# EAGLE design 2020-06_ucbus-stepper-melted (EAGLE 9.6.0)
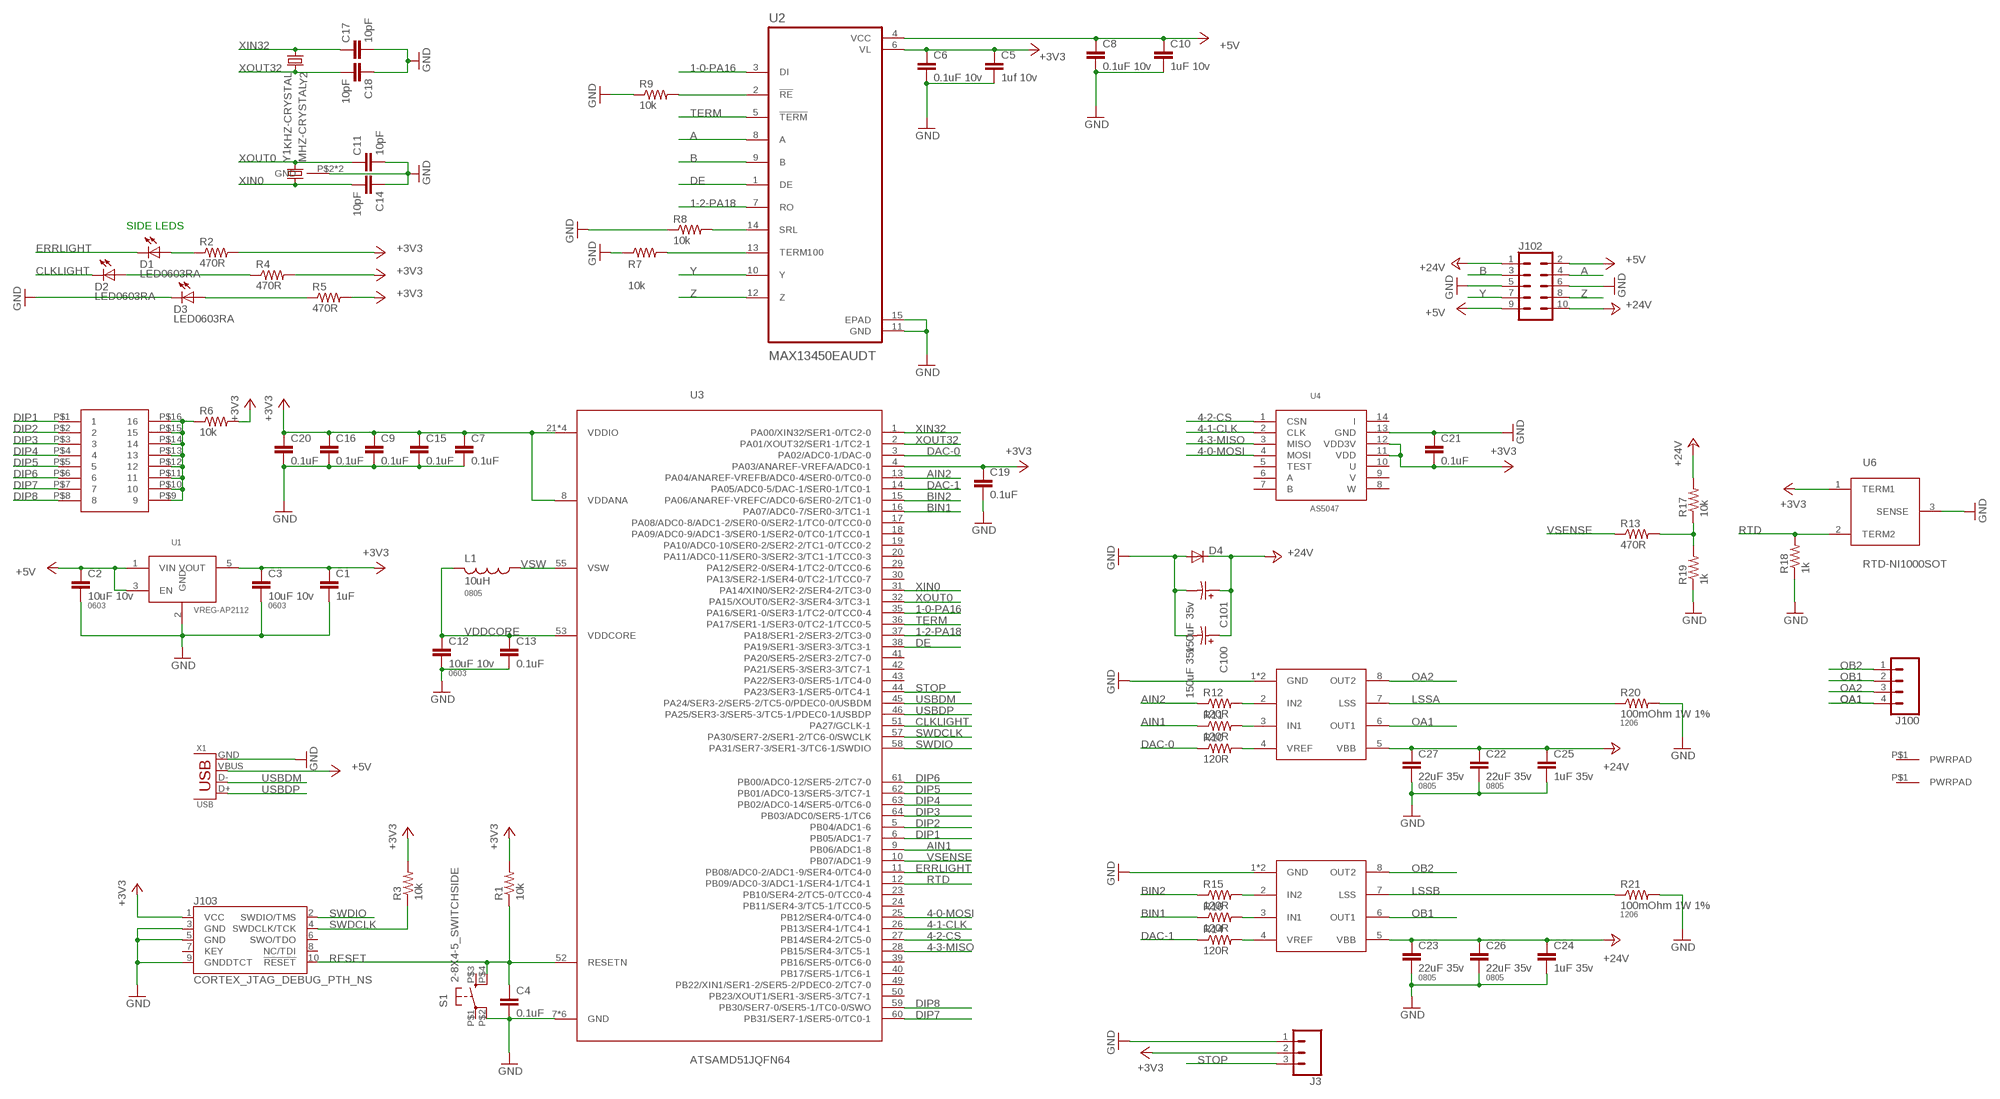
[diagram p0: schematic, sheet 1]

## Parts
C1  1uF  CAP0402  [0402]
C2  10uF 10v  CAP0603-CAP  [0603-CAP]
C3  10uF 10v  CAP0603-CAP  [0603-CAP]
C4  0.1uF  CAP0402  [0402]
C5  1uf 10v  CAP0402  [0402]
C6  0.1uF 10v  CAP0402  [0402]
C7  0.1uF  CAP0402  [0402]
C8  0.1uF 10v  CAP0402  [0402]
C9  0.1uF  CAP0402  [0402]
C10  1uF 10v  CAP0402  [0402]
C11  10pF  CAP0402  [0402]
C12  10uF 10v  CAP0603-CAP  [0603-CAP]
C13  0.1uF  CAP0402  [0402]
C14  10pF  CAP0402  [0402]
C15  0.1uF  CAP0402  [0402]
C16  0.1uF  CAP0402  [0402]
C17  10pF  CAP0402  [0402]
C18  10pF  CAP0402  [0402]
C19  0.1uF  CAP0402  [0402]
C20  0.1uF  CAP0402  [0402]
C21  0.1uF  CAP0402  [0402]
C22  22uF 35v  CAP0805  [0805]
C23  22uF 35v  CAP0805  [0805]
C24  1uF 35v  CAP0402  [0402]
C25  1uF 35v  CAP0402  [0402]
C26  22uF 35v  CAP0805  [0805]
C27  22uF 35v  CAP0805  [0805]
C100  150uF 35v  CAP-POLCAP_POL_SMD6.6X6.6  [SMD-ELEC-CAP]
C101  150uF 35v  CAP-POLCAP_POL_SMD6.6X6.6  [SMD-ELEC-CAP]
D1  LED0603RA  [LED0603-RIGHTANGLE]
D2  LED0603RA  [LED0603-RIGHTANGLE]
D3  LED0603RA  [LED0603-RIGHTANGLE]
D4  DIODESMA403D  [SMA-403D]
J1  PWRPADM3-SKINNY  [PWRPAD_3-25MM-SKINNY]
J2  PWRPADM3-SKINNY  [PWRPAD_3-25MM-SKINNY]
J3  CONN_03SMD_RA_MALE  [1X03_SMD_RA_MALE]
J100  CONN_04SCREW_LOCK  [SCREWTERMINAL-3.5MM-4_LOCK]
J101  DIPSWITCH-80100  [DIPSWITCH-8-0100]
J102  CONN_05X2SHD_LOCK_LATCH  [2X5-SHROUDED_LOCK_LATCH]
J103  CORTEX_JTAG_DEBUG_PTH_NS  [2X5-PTH-1.27MM-NO_SILK]
L1  10uH  INDUCTOR-0805  [0805]
R1  10k  RESISTOR0402  [0402]
R2  470R  RESISTOR0402  [0402]
R3  10k  RESISTOR0402  [0402]
R4  470R  RESISTOR0402  [0402]
R5  470R  RESISTOR0402  [0402]
R6  10k  RESISTOR0402  [0402]
R7  10k  RESISTOR0402  [0402]
R8  10k  RESISTOR0402  [0402]
R9  10k  RESISTOR0402  [0402]
R10  120R  RESISTOR0402  [0402]
R11  120R  RESISTOR0402  [0402]
R12  120R  RESISTOR0402  [0402]
R13  470R  RESISTOR0402  [0402]
R14  120R  RESISTOR0402  [0402]
R15  120R  RESISTOR0402  [0402]
R16  120R  RESISTOR0402  [0402]
R17  10k  RESISTOR0402  [0402]
R18  1k  RESISTOR0402  [0402]
R19  1k  RESISTOR0402  [0402]
R20  100mOhm 1W 1%  RESISTOR1206  [1206]
R21  100mOhm 1W 1%  RESISTOR1206  [1206]
S1  2-8X4-5_SWITCHSIDE  [TACT-SWITCH-SIDE]
U1  VREG-AP2112  [SOT23-5]
U2  MAX13450EAUDT  [SOP65P637X110-14N]
U3  ATSAMD51JQFN64  [QFN-64-9X9MM-SMALLPAD]
U4  AS5047  [TSSOP14]
U5  A4950  [SOIC8_PAD]
U6  RTD-NI1000SOT  [SOT23]
U7  A4950  [SOIC8_PAD]
X1  USB  [USB_MICRO_609-4613-1-ND]
Y1  MHZ-CRYSTAL  [4-SMD-3.2X2.5]
Y2  KHZ-CRYSTAL  [2-SMD-3.2X1.5MM]

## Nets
1-0-PA16: U2.3(DI) U3.35(PA16/SER1-0/SER3-1/TC2-0/TCC0-4)
1-2-PA18: U2.7(RO) U3.37(PA18/SER1-2/SER3-2/TC3-0)
4-0-MOSI: U3.25(PB12/SER4-0/TC4-0) U4.4(MOSI)
4-1-CLK: U3.26(PB13/SER4-1/TC4-1) U4.2(CLK)
4-2-CS: U3.27(PB14/SER4-2/TC5-0) U4.1(CSN)
4-3-MISO: U3.28(PB15/SER4-3/TC5-1) U4.3(MISO)
+3V3: C1.1 C3.1 C5.1 C6.1 C7.1 C9.1 C15.1 C16.1 C19.1 C20.1 C21.2 J3.2 J103.1(VCC) R1.2 R2.2 R3.2 R4.2 R5.2 R6.2 U1.5(VOUT) U2.6(VL) U3.4(PA03/ANAREF-VREFA/ADC0-1) U3.8(VDDANA) U3.21(VDDIO) U3.34(VDDIO) U3.48(VDDIO) U3.56(VDDIO) U4.11(VDD) U4.12(VDD3V) U6.1(TERM1)
+5V: C2.1 C8.1 C10.1 J102.2 J102.9 U1.1(VIN) U1.3(EN) U2.4(VCC) X1.VBUS
+24V: C22.1 C23.1 C24.1 C25.1 C26.1 C27.1 C100.A C101.A D4.P$1(C) J102.1 J102.10 R17.2 U5.5(VBB) U7.5(VBB)
A: J102.4 U2.8(A)
AIN1: R11.1 U3.9(PB06/ADC1-8)
AIN2: R12.1 U3.13(PA04/ANAREF-VREFB/ADC0-4/SER0-0/TC0-0)
B: J102.3 U2.9(B)
BIN1: R16.1 U3.16(PA07/ADC0-7/SER0-3/TC1-1)
BIN2: R15.1 U3.15(PA06/ANAREF-VREFC/ADC0-6/SER0-2/TC1-0)
CLKLIGHT: D2.2(C) U3.51(PA27/GCLK-1)
DAC-0: R10.1 U3.3(PA02/ADC0-1/DAC-0)
DAC-1: R14.1 U3.14(PA05/ADC0-5/DAC-1/SER0-1/TC0-1)
DE: U2.1(DE) U3.38(PA19/SER1-3/SER3-3/TC3-1)
DIP1: J101.P$1 U3.6(PB05/ADC1-7)
DIP2: J101.P$2 U3.5(PB04/ADC1-6)
DIP3: J101.P$3 U3.64(PB03/ADC0/SER5-1/TC6)
DIP4: J101.P$4 U3.63(PB02/ADC0-14/SER5-0/TC6-0)
DIP5: J101.P$5 U3.62(PB01/ADC0-13/SER5-3/TC7-1)
DIP6: J101.P$6 U3.61(PB00/ADC0-12/SER5-2/TC7-0)
DIP7: J101.P$7 U3.60(PB31/SER7-1/SER5-0/TC0-1)
DIP8: J101.P$8 U3.59(PB30/SER7-0/SER5-1/TC0-0/SWO)
ERRLIGHT: D1.2(C) U3.11(PB08/ADC0-2/ADC1-9/SER4-0/TC4-0)
GND: C1.2 C2.2 C3.2 C4.2 C5.2 C6.2 C7.2 C8.2 C9.2 C10.2 C11.2 C12.2 C13.2 C14.1 C15.2 C16.2 C17.2 C18.1 C19.2 C20.2 C21.1 C22.2 C23.2 C24.2 C25.2 C26.2 C27.2 C100.C C101.C D3.2(C) D4.P$2(A) J3.1 J102.5 J102.6 J103.3(GND) J103.5(GND) J103.9(GNDDTCT) R7.1 R8.1 R9.1 R18.1 R19.1 R20.2 R21.2 S1.P$2(P1) U1.2(GND) U2.11(GND) U2.15(EPAD) U3.7(GND) U3.22(GND) U3.33(GND) U3.47(GND) U3.54(GND) U3.P$1(GND) U4.13(GND) U5.1(GND) U5.P$1(GND) U6.3(SENSE) U7.1(GND) U7.P$1(GND) X1.GND Y1.P$2(GND) Y1.P$4(GND)
LSSA: R20.1 U5.7(LSS)
LSSB: R21.1 U7.7(LSS)
N$1: R11.2 U5.3(IN1)
N$2: R14.2 U7.4(VREF)
N$3: R10.2 U5.4(VREF)
N$4: R12.2 U5.2(IN2)
N$5: D3.1(A) R5.1
N$6: J101.P$9 J101.P$10 J101.P$11 J101.P$12 J101.P$13 J101.P$14 J101.P$15 J101.P$16 R6.1
N$7: R15.2 U7.2(IN2)
N$8: R16.2 U7.3(IN1)
N$9: D2.1(A) R4.1
N$10: D1.1(A) R2.1
N$11: R9.2 U2.2(!RE)
N$17: R13.2 R17.1 R19.2
N$18: R7.2 U2.13(TERM100)
N$19: R8.2 U2.14(SRL)
OA1: J100.4 U5.6(OUT1)
OA2: J100.3 U5.8(OUT2)
OB1: J100.2 U7.6(OUT1)
OB2: J100.1 U7.8(OUT2)
RESET: C4.1 J103.10(!RESET) R1.1 S1.P$4(S1) U3.52(RESETN)
RTD: R18.2 U3.12(PB09/ADC0-3/ADC1-1/SER4-1/TC4-1) U6.2(TERM2)
STOP: J3.3 U3.44(PA23/SER3-1/SER5-0/TC4-1)
SWDCLK: J103.4(SWDCLK/TCK) R3.1 U3.57(PA30/SER7-2/SER1-2/TC6-0/SWCLK)
SWDIO: J103.2(SWDIO/TMS) U3.58(PA31/SER7-3/SER1-3/TC6-1/SWDIO)
TERM: U2.5(!TERM) U3.36(PA17/SER1-1/SER3-0/TC2-1/TCC0-5)
USBDM: U3.45(PA24/SER3-2/SER5-2/TC5-0/PDEC0-0/USBDM) X1.D-
USBDP: U3.46(PA25/SER3-3/SER5-3/TC5-1/PDEC0-1/USBDP) X1.D+
VDDCORE: C12.1 C13.1 L1.2 U3.53(VDDCORE)
VSENSE: R13.1 U3.10(PB07/ADC1-9)
VSW: L1.1 U3.55(VSW)
XIN0: C14.2 U3.31(PA14/XIN0/SER2-2/SER4-2/TC3-0) Y1.P$1
XIN32: C17.1 U3.1(PA00/XIN32/SER1-0/TC2-0) Y2.P$1
XOUT0: C11.1 U3.32(PA15/XOUT0/SER2-3/SER4-3/TC3-1) Y1.P$3
XOUT32: C18.2 U3.2(PA01/XOUT32/SER1-1/TC2-1) Y2.P$2
Y: J102.7 U2.10(Y)
Z: J102.8 U2.12(Z)
Unconnected: J1.P$1(PWRPAD) J2.P$1(PWRPAD) J103.6(SWO/TDO) J103.7(KEY) J103.8(NC/TDI) S1.P$1(P) S1.P$3(S) U3.17(PA08/ADC0-8/ADC1-2/SER0-0/SER2-1/TC0-0/TCC0-0) U3.18(PA09/ADC0-9/ADC1-3/SER0-1/SER2-0/TC0-1/TCC0-1) U3.19(PA10/ADC0-10/SER0-2/SER2-2/TC1-0/TCC0-2) U3.20(PA11/ADC0-11/SER0-3/SER2-3/TC1-1/TCC0-3) U3.23(PB10/SER4-2/TC5-0/TCC0-4) U3.24(PB11/SER4-3/TC5-1/TCC0-5) U3.29(PA12/SER2-0/SER4-1/TC2-0/TCC0-6) U3.30(PA13/SER2-1/SER4-0/TC2-1/TCC0-7) U3.39(PB16/SER5-0/TC6-0) U3.40(PB17/SER5-1/TC6-1) U3.41(PA20/SER5-2/SER3-2/TC7-0) U3.42(PA21/SER5-3/SER3-3/TC7-1) U3.43(PA22/SER3-0/SER5-1/TC4-0) U3.49(PB22/XIN1/SER1-2/SER5-2/PDEC0-2/TC7-0) U3.50(PB23/XOUT1/SER1-3/SER5-3/TC7-1) U4.5(TEST) U4.6(A) U4.7(B) U4.8(W) U4.9(V) U4.10(U) U4.14(I)

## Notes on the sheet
- SIDE LEDS

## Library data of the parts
C1 C4-C11 C13-C21 C24 C25 = passives:CAP: Capacitor
C2 C3 C12 = passives:CAP: Capacitor; PACKAGE: 0603
C22 C23 C26 C27 = passives:CAP: Capacitor; PACKAGE: 0805
C100 C101 = passives:CAP-POL
D1-D3 = lights:LED: LED
D4 = passives:DIODE: DIODE
J1 J2 = connector:PWRPAD
J3 = SparkFun-Connectors:CONN_03: Multi connection point. Often used as Generic Header-pin footprint for 0.1 inch spaced/style header connections On any of the 0.1 inch spaced packages, you can populate with these: Break Away Headers - Straight (PRT-00116) Break Away Male Headers - Right Angle (PRT-00553) Female Headers (PRT-00115)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; PROD_ID: CONN-10925
J100 = SparkFun-Connectors:CONN_04: Multi connection point. Often used as Generic Header-pin footprint for 0.1 inch spaced/style header connections On any of the 0.1 inch spaced packages, you can populate with these: Break Away Headers - Straight (PRT-00116) Break Away Male Headers - Right Angle (PRT-00553) Female Headers (PRT-00115)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
J101 = passives:DIPSWITCH-8
J102 = SparkFun-Connectors:CONN_05X2: Multi connection point. Often used as Generic Header-pin footprint for 0.1 inch spaced/style header connections For AVR SPI programming port, see special device with nice symbol: "AVR_SPI_PROG_5x2.dev" You can populate with any combo of single row headers, but if you'd like an exact match, check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
J103 = SparkFun-Connectors:CORTEX_JTAG_DEBUG: Cortex Debug Connector - 10 pin Supports JTAG debug, Serial Wire debug, and Serial Wire Viewer. PTH and SMD connector options available. General Connector Information Products: PTH Connector -via Digi-Key SparkFun PSoc SparkFun T
L1 = passives:INDUCTOR; PACKAGE: 0805
R1-R19 = passives:RESISTOR: Resistor
R20 R21 = passives:RESISTOR: Resistor; PACKAGE: 1206
S1 = passives:2-8X4-5_SWITCH
U1 = power:VREG-AP2112
U2 = comm:MAX13450EAUDT; DESCRIPTION: 1/1 Transceiver Full RS422, RS485 14-TSSOP-EP; DIGI-KEY_PART_NUMBER: MAX13450EAUD+T-ND; DIGIKEY-PURCHASE-URL: https://snapeda.com/shop?store=DigiKey&id=694117; MF: Maxim Integrated; MP: MAX13450EAUD+; PACKAGE: TSSOP-14 Maxim
U3 = microcontrollers:ATSAMD51J
U4 = sensor:AS5047
U5 U7 = power:A4950
U6 = sensor:RTD-NI1000SOT
X1 = connector:USB: SMD micro USB connector as found in the fablab inventory. Three footprint variants included: 609-4613-1-ND used by Jake original, as described by manufacturer's datasheet for milling with the 1/100" bit for milling with the 1/64" bit Made by Zaerc.
Y1 = passives:MHZ-CRYSTAL
Y2 = passives:KHZ-CRYSTAL

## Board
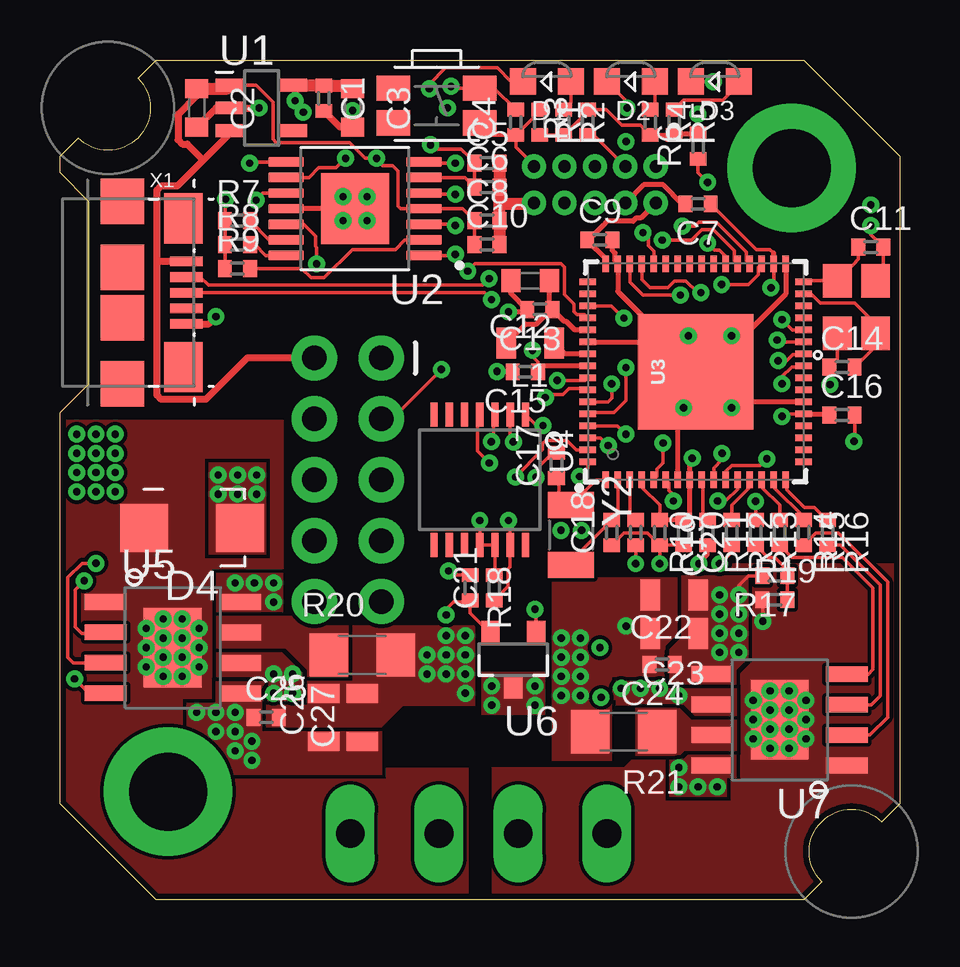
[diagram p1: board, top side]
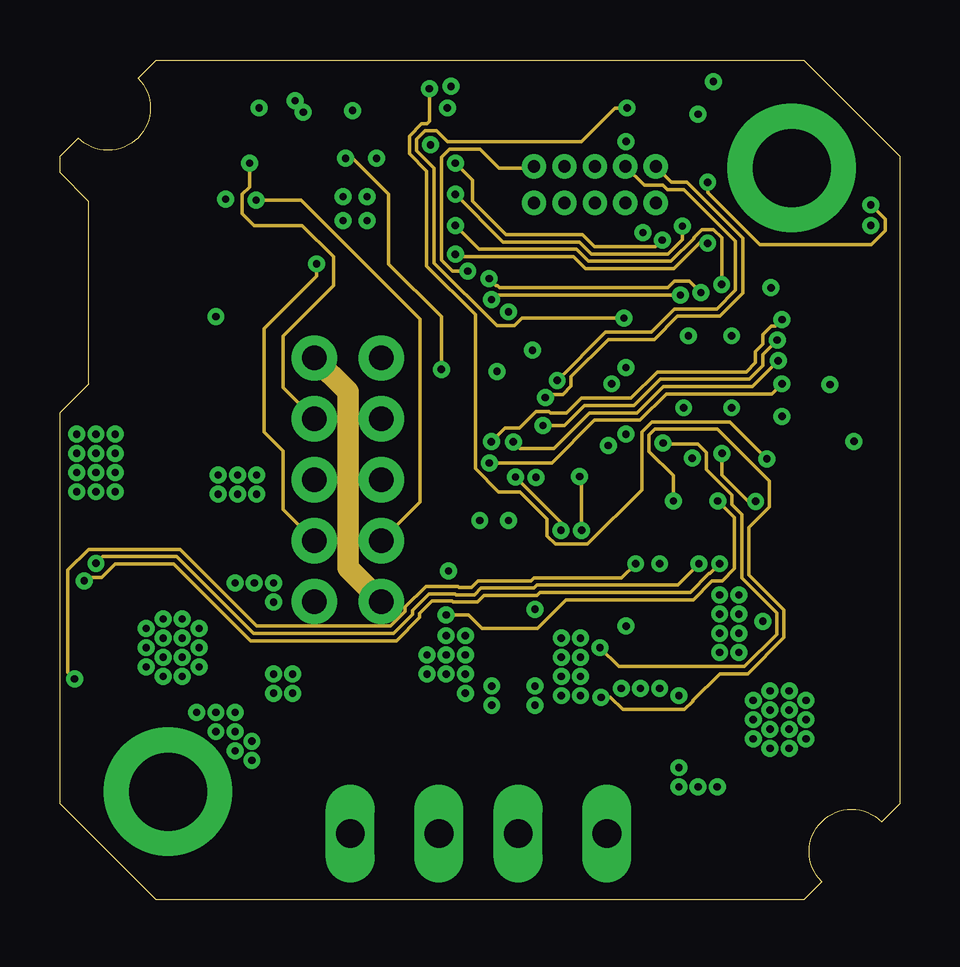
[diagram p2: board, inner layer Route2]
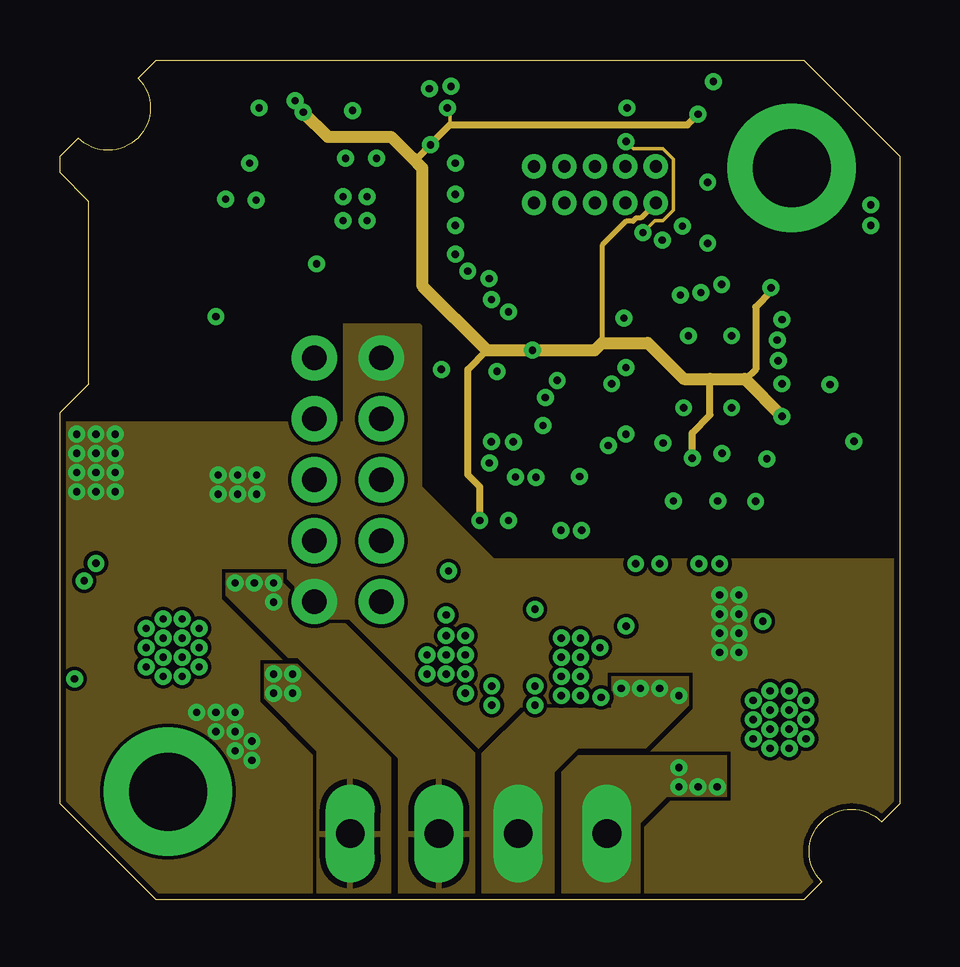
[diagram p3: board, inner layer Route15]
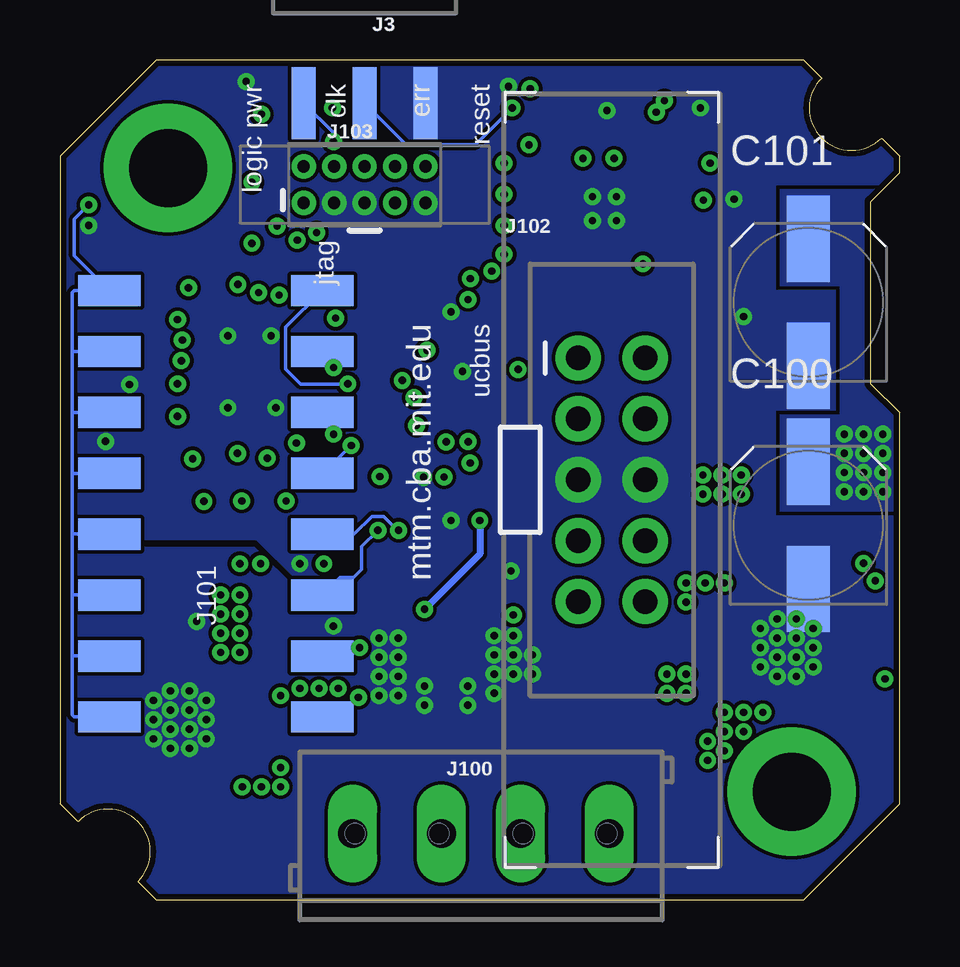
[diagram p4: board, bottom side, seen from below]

Size 35 x 35 mm. Coordinates in mm from the lower left corner, seen from the top.
Outline: 31,35 35,31 35,4 34.25,3.25 arc180 31.75,0.75 31,0 4,0 0,4 0,20.3 1.2,21.5 1.2,29.1 0,30.3 0,31 0.75,31.75 arc180 3.25,34.25 4,35 31,35
Copper layers (1+2*15+16): Top 0.035mm / dielectric 1.5mm / Route2 0.035mm / dielectric 0.15mm / Route15 0.035mm / dielectric 0.2mm / Bottom 0.035mm
Design rules "default *": minimum track width 6mil, minimum drill 10mil, track to track 6mil, track to pad 6mil, pad to pad 6mil, via to via 6mil, smd to smd 0mil, copper to edge 10mil, drill to drill 6mil, minimum pad ring 10mil, minimum via ring 8mil, stop-mask expansion 4mil, vias tented up to drill 35mil, thermal gap 10mil

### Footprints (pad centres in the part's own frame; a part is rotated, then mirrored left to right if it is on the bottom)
0402 = smd 0.575 x 0.7: 1 -0.525,0; 2 0.525,0
0603-CAP = smd 0.8 x 0.95: 1 -0.8,0; 2 0.8,0
0805 = smd 0.8 x 1.3: 1 -1,0; 2 1,0
SMD-ELEC-CAP = smd 1.8 x 3.6: A 0,2.65; C 0,-2.65
LED0603-RIGHTANGLE = smd 1.1 x 1.1: 1 -1,0; 2 1,0
SMA-403D = smd 2 x 2: P$1 -2,0; P$2 2,0
PWRPAD_3-25MM-SKINNY = drill 3.25 pad 5.35: P$1 0,0
1X03_SMD_RA_MALE = smd 1 x 3: 1 -2.54,5; 2 0,5; 3 2.54,5
SCREWTERMINAL-3.5MM-4_LOCK = drill 1.2 pad 2.032 long: 1 -0.1,0; 2 3.6,0; 3 6.9,0; 4 10.6,0
DIPSWITCH-8-0100 = smd 1.3 x 2.6: P$1 -8.89,-4.445; P$2 -6.35,-4.445; P$3 -3.81,-4.445; P$4 -1.27,-4.445; P$5 1.27,-4.445; P$6 3.81,-4.445; P$7 6.35,-4.445; P$8 8.89,-4.445; P$9 8.89,4.445; P$10 6.35,4.445; P$11 3.81,4.445; P$12 1.27,4.445; P$13 -1.27,4.445; P$14 -3.81,4.445; P$15 -6.35,4.445; P$16 -8.89,4.445
2X5-SHROUDED_LOCK_LATCH = drill 1.016 pad 1.88: 1 -1.397,5.08; 2 1.397,5.08; 3 -1.397,2.54; 4 1.397,2.54; 5 -1.397,0; 6 1.397,0; 7 -1.397,-2.54; 8 1.397,-2.54; 9 -1.397,-5.08; 10 1.397,-5.08
2X5-PTH-1.27MM-NO_SILK = drill 0.508 pad 1: 1 -2.54,-0.762; 2 -2.54,0.762; 3 -1.27,-0.762; 4 -1.27,0.762; 5 0,-0.762; 6 0,0.762; 7 1.27,-0.762; 8 1.27,0.762; 9 2.54,-0.762; 10 2.54,0.762
1206 = smd 1.6 x 1.8: 1 -1.4,0; 2 1.4,0
TACT-SWITCH-SIDE = smd 1.4 x 1.05: P$1 -1.8,0.725; P$2 1.8,0.725; P$3 -1.8,-0.725; P$4 1.8,-0.725
SOT23-5 = smd 0.533 x 1.194: 1 -0.95,-1.306; 2 0,-1.306; 3 0.95,-1.306; 4 0.95,1.306; 5 -0.95,1.306
SOP65P637X110-14N = smd 1.48 x 0.41: 1 -2.875,1.95; 2 -2.875,1.3; 3 -2.875,0.65; 4 -2.875,0; 5 -2.875,-0.65; 6 -2.875,-1.3; 7 -2.875,-1.95; 8 2.875,-1.95; 9 2.875,-1.3; 10 2.875,-0.65; 11 2.875,0; 12 2.875,0.65; 13 2.875,1.3; 14 2.875,1.95 | smd 2.85 x 2.95: 15 0,0
QFN-64-9X9MM-SMALLPAD = smd 0.7 x 0.275: 1 -4.5,3.75; 2 -4.5,3.25; 3 -4.5,2.75; 4 -4.5,2.25; 5 -4.5,1.75; 6 -4.5,1.25; 7 -4.5,0.75; 8 -4.5,0.25; 9 -4.5,-0.25; 10 -4.5,-0.75; 11 -4.5,-1.25; 12 -4.5,-1.75; 13 -4.5,-2.25; 14 -4.5,-2.75; 15 -4.5,-3.25; 16 -4.5,-3.75; 33 4.5,-3.75; 34 4.5,-3.25; 35 4.5,-2.75; 36 4.5,-2.25; 37 4.5,-1.75; 38 4.5,-1.25; 39 4.5,-0.75; 40 4.5,-0.25; 41 4.5,0.25; 42 4.5,0.75; 43 4.5,1.25; 44 4.5,1.75; 45 4.5,2.25; 46 4.5,2.75; 47 4.5,3.25; 48 4.5,3.75 | smd 0.275 x 0.7: 17 -3.75,-4.5; 18 -3.25,-4.5; 19 -2.75,-4.5; 20 -2.25,-4.5; 21 -1.75,-4.5; 22 -1.25,-4.5; 23 -0.75,-4.5; 24 -0.25,-4.5; 25 0.25,-4.5; 26 0.75,-4.5; 27 1.25,-4.5; 28 1.75,-4.5; 29 2.25,-4.5; 30 2.75,-4.5; 31 3.25,-4.5; 32 3.75,-4.5; 49 3.75,4.5; 50 3.25,4.5; 51 2.75,4.5; 52 2.25,4.5; 53 1.75,4.5; 54 1.25,4.5; 55 0.75,4.5; 56 0.25,4.5; 57 -0.25,4.5; 58 -0.75,4.5; 59 -1.25,4.5; 60 -1.75,4.5; 61 -2.25,4.5; 62 -2.75,4.5; 63 -3.25,4.5; 64 -3.75,4.5 | smd 4.8 x 4.8: P$1 0,0
TSSOP14 = smd 0.305 x 0.991: 1 -1.905,-2.718; 2 -1.27,-2.718; 3 -0.635,-2.718; 4 0,-2.718; 5 0.635,-2.718; 6 1.27,-2.718; 7 1.905,-2.718; 8 1.905,2.718; 9 1.27,2.718; 10 0.635,2.718; 11 0,2.718; 12 -0.635,2.718; 13 -1.27,2.718; 14 -1.905,2.718
SOIC8_PAD = smd 1.75 x 0.65: 1 -2.8,1.905; 2 -2.8,0.645; 3 -2.8,-0.625; 4 -2.8,-1.895; 5 2.8,-1.905; 6 2.8,-0.635; 7 2.8,0.635; 8 2.8,1.905 | smd 2.41 x 3.3: P$1 0,0
SOT23 = smd 0.762 x 1.016: 1 -0.95,-1.1; 2 0.95,-1.1; 3 0,1.1
USB_MICRO_609-4613-1-ND = smd 0.4 x 1.35: D+ 0,2.675; D- -0.65,2.675; GND 1.3,2.675; ID 0.65,2.675; VBUS -1.3,2.675 | smd 1.9 x 1.8: HD0 -3.8,0; HD1 -1.05,0; HD2 1.05,0; HD3 3.8,0 | smd 2.1 x 1.6: HD4 -3.1,2.55; HD5 3.1,2.55
4-SMD-3.2X2.5 = smd 1.4 x 1.2: P$1 -1.1,-0.8; P$2 1.1,-0.8; P$3 1.1,0.8; P$4 -1.1,0.8
2-SMD-3.2X1.5MM = smd 1.1 x 1.9: P$1 -1.25,0; P$2 1.25,0

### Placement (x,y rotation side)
C1  11,33.4 270 top
C2  5.7,33 270 top
C3  12.2,33 270 top
C4  19,32.4 90 top
C5  17.8,30.7 0 top
C6  17.8,29.7 0 top
C7  26.6,29 180 top
C8  17.8,28.3 0 top
C9  22.5,27.5 0 top
C10  17.8,27.3 0 top
C11  33.8,27.2 0 top
C12  19.6,25.8 180 top
C13  20,24.6 180 top
C14  32.6,22.2 0 top
C15  19.4,22 180 top
C16  32.6,20.2 0 top
C17  20.7,18.1 90 top
C18  23,15.3 90 top
C19  25,15.3 270 top
C20  26,15.3 270 top
C21  18.1,13 90 top
C22  25.6,12.7 180 top
C23  25.6,11.1 180 top
C24  25.1,9.8 180 top
C25  8.6,7.6 0 top
C26  11,7.6 90 top
C27  12.6,7.6 90 top
C100  3.8,15.6 0 bottom
C101  3.8,24.9 0 bottom
D1  20.3,34.1 180 top
D2  23.8,34.1 180 top
D3  27.3,34.1 180 top
D4  5.5,15.5 180 top
J1  30.5,30.5 0 top
J2  4.5,4.5 0 top
J3  22.3,38.2 180 bottom
J100  22.7,2.75 0 bottom
J101  28.5,16.5 90 bottom
J102  12,17.5 0 bottom
J103  22.3,29.8 0 bottom
L1  19.6,23.2 180 top
R1  20,32.4 270 top
R2  21,32.4 270 top
R3  22,32.4 90 top
R4  24.6,32.4 270 top
R5  25.6,32.4 270 top
R6  26.6,31.4 90 top
R7  7.4,28.3 0 top
R8  7.4,27.3 0 top
R9  7.4,26.3 0 top
R10  24,15.3 270 top
R11  27,15.3 270 top
R12  28,15.3 270 top
R13  29,15.3 270 top
R14  30,15.3 270 top
R15  31,15.3 270 top
R16  32,15.3 270 top
R17  29.8,13.5 180 top
R18  17.1,13 270 top
R19  29.8,12.5 0 top
R20  12.6,10.2 0 top
R21  23.5,7 180 top
S1  15.7,33.1 0 top
U1  8.4,33 270 top
U2  12.3,28.8 180 top
U3  26.5,22 90 top
U4  17.5,17.5 180 top
U5  4.7,10.5 0 top
U6  18.9,10 180 top
U7  30,7.5 180 top
X1  2.6,25.3 270 top
Y1  33.2,24.7 90 top
Y2  21.3,15.2 270 top

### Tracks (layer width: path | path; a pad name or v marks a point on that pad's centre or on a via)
1-0-PA16  (via drill 0.3)
  Top 0.152: U2.3 16.43,28.15 v16.48,28.1 | U3.35 29.12,26.37 29.12,26.05 28.7,25.64 v27.58,25.64
  Route2 0.152: v16.48,28.1 17.48,27.11 21.53,27.11 22.03,26.61 25.47,26.61 26.42,27.55 26.42,27.6 26.76,27.94 27.24,27.94 27.58,27.59 v27.58,25.64
1-2-PA18  (via drill 0.3)
  Top 0.152: U2.7 15.23,30.7 v16.48,30.7 | U3.37 28.12,26.63 28.12,27.06 27.24,27.94 26.76,27.94 26.31,27.49 v25.11,27.49
  Route2 0.152: v16.48,30.7 17.2,29.98 17.2,29.11 18.6,27.71 21.78,27.71 22.28,27.21 24.83,27.21 v25.11,27.49
4-0-MOSI  (via drill 0.3)
  Top 0.152: U3.25 30.95,22.2 30.5,22.2 30.1,21.8 v30.1,21.5 | v17.9,18.2 17.4,18.7 17.4,20.12 U4.4
  Route2 0.152: v30.1,21.5 29.68,21.08 25.28,21.08 24.18,19.98 22.28,19.98 20.5,18.2 v17.9,18.2
4-1-CLK  (via drill 0.3)
  Top 0.152: U3.26 30.97,22.72 30.55,22.72 30.3,22.46 v29.94,22.46 | v18.9,19.08 18.77,19.21 U4.2
  Route2 0.152: v29.94,22.46 28.86,21.39 25.16,21.39 24.06,20.29 22.08,20.29 20.6,18.8 19.18,18.8 v18.9,19.08
4-2-CS  (via drill 0.3)
  Top 0.152: U3.27 29.97,23.25 v29.9,23.32 | v20.14,19.76 19.86,19.76 U4.1
  Route2 0.152: v29.9,23.32 29.3,22.72 29.3,22.25 28.74,21.69 25.03,21.69 23.93,20.59 21.86,20.59 21.03,19.76 v20.14,19.76
4-3-MISO  (via drill 0.3)
  Top 0.152: U3.28 30.53,23.75 v30.1,24.18 | v17.98,19.09 18.08,19.18 18.08,20.16 U4.3
  Route2 0.152: v30.1,24.18 29.82,23.9 29.66,23.9 29.3,23.54 29.3,23.15 29,22.85 29,22.38 28.61,22 24.9,22 23.8,20.9 21.73,20.9 21.12,20.28 20.44,20.28 20.38,20.35 19.85,20.35 19.16,19.66 18.56,19.66 v17.98,19.09
+3V3  (via drill 0.3)
  Top 0.152: C21.2 18.14,13.56 U4.12 U4.11 v17.5,15.8 | U6.1 19.85,12.05 v19.8,12.1 | U3.4 24.28,17.47 24.28,17.16 25,16.44 C19.1 | U3.21 30.4,20.25 30.29,20.14 v30.1,20.14 | U3.34 29.75,25.61 v29.64,25.5 | C9.1 22.03,27.5 | U2.6 16.88,30.1 C6.1 C5.1 17.06,30.91 17.06,30.94 16.72,31.28 15.63,31.28 v15.45,31.46 | R1.2 R2.2 22,32.88 R3.2 22.77,32.92 23.43,32.27 24.2,32.27 R4.2 | C15.1 19.93,22.4 19.69,22.63 v19.69,22.9 | C7.1 29.02,27.1 29.6,27.1 29.75,26.95
  Top 0.203: U3.56 20.18,22.25 C15.1 | U3.21 32.02,20.25 C16.1 | U3.34 29.75,26.95 | C9.1 22.75,26.73 U3.48 | v26.36,18.4 26.25,18.29 U3.8 26.25,16.07 C20.1 C19.1 | R4.2 R5.2 25.65,31.92 R6.2 v26.6,32.74 | 22.03,27.5 22.48,27.95 22.63,28.1 22.64,28.1 22.81,28.28 23.89,28.28 24.02,28.41 24.21,28.41 J103.1
  Top 0.3: U1.5 9.8,33.86 v9.8,33.3 10.14,32.96 v10.14,32.82
  Top 0.5: U1.5 10.97,33.95 C1.1 12.07,33.92 C3.1
  Route15 0.152: v16.15,33 16.25,32.9 16.25,32.3
  Route15 0.203: J103.1 24.21,28.41 24.02,28.41 23.89,28.28 23.6,28.28 22.6,27.28 22.6,23.2
  Route15 0.3: v29.64,25.5 29.64,25.34 29,24.7 29,22.1 28.57,21.67 | v26.36,18.4 26.36,19.46 27.1,20.2 27.1,21.7 | v17.5,15.8 17.5,17.2 17,17.7 17,22.1 17.8,22.9 | 14.65,30.95 14.94,30.95 v15.45,31.46 15.45,31.5 16.25,32.3 26.16,32.3 v26.6,32.74
  Route15 0.5: v10.14,32.82 11.17,31.8 13.8,31.8 14.65,30.95 15.1,30.5 15.1,25.6 17.8,22.9 v19.69,22.9 22.3,22.9 22.6,23.2 24.5,23.2 26,21.7 27.1,21.7 28.54,21.7 28.57,21.67 v30.1,20.14
  Bottom 0.152: J3.2 20.57,31.47 17.68,31.47 v16.15,33
  Bottom 0.3: v17.5,15.8 17.5,14.4 v19.8,12.1
+5V  (via drill 0.3)
  Top 0.152: C10.1 C8.1 16.77,28.8 U2.4 14.2,28.8 14.1,28.9 14.1,30.37 13.87,30.6 13.45,30.6 13.2,30.85 v13.2,30.9 12.72,30.9 12.07,31.55 9.01,31.55 8.88,31.69 8.88,32.76 8.88,33.24 8.17,33.95 U1.1
  Top 0.3: J102.2 7.81,22.58 6.07,20.85 4.22,20.85 4.05,21.02 4.05,26.6 | 5.97,30.83 4.9,29.75 4.22,29.75 4.05,29.58 4.05,26.6 | 5.97,30.83 7.09,31.95 U1.3 | X1.VBUS 4.05,26.6 | C2.1 5.7,33.5 4.92,32.73 4.92,31.67 5.1,31.5 5.3,31.5 5.97,30.83
  Top 0.5: C2.1 6.94,33.8 U1.1
  Route2 0.9: J102.9 12,13.82 12,21.18 J102.2
+24V  (via drill 0.3)
  Top 0.152: v28.3,12.7 28.3,13.1 28.7,13.5 R17.2
  other vias: 27.5,12.7 28.3,11.9 28.3,11.1 28.3,10.3 27.5,10.3 27.5,11.1 27.5,11.9 7.3,7.8 7.3,7 7.3,6.2 6.5,7.8 6.5,7 5.7,7.8 8,5.8 8,6.6 2.3,17 2.3,17.8 2.3,18.6 2.3,19.4 1.5,17 1.5,17.8 1.5,18.6 1.5,19.4 0.7,19.4 0.7,18.6 0.7,17.8 0.7,17 8.2,16.9 7.4,16.9 6.6,16.9 6.6,17.7 7.4,17.7 8.2,17.7
  pour Top (rank 3, no thermals): 28.2,9 28.2,9.6 28.7,10.1 28.7,13.5 25.9,13.5 25.9,10.9 25.4,10.4 25.4,9
  pour Route15 (rank 6, no thermals): 36.5,14.2 18.1,14.2 15.1,17.2 15.1,23.9 15,24 11.8,24 11.8,19.9 -1.5,19.9 -1.5,-1.5 36.5,-1.5
  pour Top (rank 4, no thermals): 6.5,9.1 8.5,9.1 8.5,7.1 13.4,7.1 13.4,5.2 6.7,5.2 6.7,5.4 5.3,6.8 5.3,8.2 6.5,8.2
  pour Bottom (rank 4, no thermals): 5,29.6 5,25.6 2.5,25.6 2.5,20.2 5,20.2 5,16.2 -2,16.2 -2,29.6
  pour Top (rank 4, no thermals): 8.6,14.4 8.6,18.2 6.2,18.2 6.2,14.4
A  (via drill 0.3)
  Top 0.152: U2.8 7.95,30.75 v7.9,30.7
  Route2 0.152: v7.9,30.7 7.9,29.7 7.6,29.4 7.6,28.6 8.1,28.1 10.1,28.1 11.4,26.8 11.4,25.6 9.3,23.5 9.3,21.34 J102.4
AIN1
  Top 0.152: U3.9 26.8,17.45 26.8,16.02 R11.1
AIN2
  Top 0.152: U3.13 28.72,17.47 28.72,17.16 28,16.44 R12.1
B  (via drill 0.3)
  Top 0.152: J102.3 13.84,20.04 v15.9,22.1 | v11.9,30.9 11.5,30.5 10.78,30.5 10.38,30.1 U2.9
  Route2 0.152: v15.9,22.1 15.9,24.3 13.7,26.5 13.7,29.4 12.2,30.9 v11.9,30.9
BIN1
  Top 0.152: U3.16 30.3,17.45 30.3,17.07 31.03,16.34 31.45,16.34 31.96,15.82 R16.1
BIN2
  Top 0.152: U3.15 29.78,17.47 29.78,17.16 31,15.94 R15.1
CLKLIGHT  (via drill 0.3)
  Top 0.152: D2.2 23.64,33.26 v23.64,33 | U3.51 22.99,24.75 v23.51,24.23
  Route2 0.152: v23.51,24.23 19.26,24.23 18.94,23.92 18.21,23.92 15.59,26.53 15.59,30.49 14.87,31.22 14.87,31.7 15.21,32.04 15.69,32.04 16.15,31.59 21.73,31.59 23.14,33 v23.64,33
DAC-0
  Top 0.152: U3.3 23.75,16.07 R10.1
DAC-1
  Top 0.152: U3.14 29.28,17.47 29.28,17.16 30,16.44 R14.1
DE  (via drill 0.3)
  Top 0.152: U2.1 16.43,26.85 v16.48,26.9 | v27,27.36 27.28,27.08 27.48,27.08 27.75,26.81 U3.38
  Route2 0.152: v16.48,26.9 16.58,26.8 21.4,26.8 21.9,26.3 25.6,26.3 26.66,27.36 v27,27.36
DIP1  (via drill 0.3)
  Top 0.152: U3.6 25.38,17.37 25.38,17.05 25.57,16.87 v25.57,16.62
  Route2 0.152: v22.56,8.43 22.95,8.43 23.46,7.92 26.04,7.92 26.38,8.26 26.38,8.29 27.5,9.41 28.67,9.41 30.19,10.93 30.19,12.07 28.73,13.53 28.73,15.5 29.58,16.36 29.58,17.44 27.41,19.61 24.8,19.61 24.56,19.37 24.56,18.68 25.57,17.68 v25.57,16.62
  Bottom 0.152: J101.P$1 23.38,7.61 v22.56,8.43
DIP2  (via drill 0.3)
  Top 0.152: U3.5 24.88,17.63 24.88,17.95 25.14,18.2 v25.14,19.03
  Route2 0.152: v22.52,10.5 23.3,9.72 28.54,9.72 29.88,11.06 29.88,11.94 28.42,13.4 28.42,16.04 28,16.47 28,16.86 26.94,17.92 26.94,18.64 26.6,18.98 25.19,18.98 v25.14,19.03
  Bottom 0.152: J101.P$2 22.86,10.15 v22.52,10.5
DIP3  (via drill 0.3)
  Top 0.152: U3.64 22,17.97 v21.66,17.64
  Route2 0.152: v21.75,15.39 21.75,17.55 v21.66,17.64
  Bottom 0.152: J101.P$3 23.33,13.42 22.76,13.42 22.42,13.76 22.42,14.72 v21.75,15.39
DIP4  (via drill 0.3)
  Top 0.152: v18.99,17.62 20.12,18.75 20.12,19.01 20.25,19.14 21.14,19.14 21.54,18.75 U3.63
  Route2 0.152: v20.89,15.39 20.89,15.72 v18.99,17.62
  Bottom 0.152: J101.P$4 22.73,15.23 21.99,15.98 21.51,15.98 20.92,15.39 v20.89,15.39
DIP5  (via drill 0.3)
  Top 0.152: U3.62 22.53,19.25 v22.86,18.92
  Bottom 0.152: v22.86,18.92 24.01,17.77 J101.P$5
DIP6  (via drill 0.3)
  Top 0.152: U3.61 23.24,19.75 v23.59,19.4
  Bottom 0.152: v23.59,19.4 23.59,19.85 J101.P$6
DIP7  (via drill 0.3)
  Top 0.152: U3.60 22.05,20.3 23.1,20.3 23.59,20.79 v23.59,22.18
  Bottom 0.152: v23.59,22.18 24.05,22.64 J101.P$7
DIP8  (via drill 0.3)
  Top 0.152: U3.59 22.85,20.75 23,20.9 v23,21.5
  Bottom 0.152: v23,21.5 24.98,21.5 25.58,22.11 25.58,23.86 J101.P$8
ERRLIGHT  (via drill 0.3)
  Top 0.152: v29.47,18.37 29.2,18.1 28.01,18.1 27.76,17.86 U3.11 | D1.2 18.8,34.1 18.23,34.67 16.07,34.67 15.4,34 v15.4,33.8
  Route2 0.152: v29.47,18.37 27.93,19.91 24.68,19.91 24.26,19.49 24.26,17.08 21.99,14.81 20.65,14.81 20.31,15.15 20.31,15.87 19.17,17 18.28,17 17.32,17.96 17.32,24.38 15.29,26.41 15.29,30.37 14.56,31.09 14.56,31.83 15.08,32.35 15.3,32.35 15.4,32.45 v15.4,33.8
GND  (via drill 0.3)
  Top 0.152: R19.1 29.3,12.47 v29.3,11.6 | U3.P$1 26.4,21.9 26.4,22.2 | C21.1 18.68,13.05 18.68,13.78 18.77,13.87 U4.13 18.77,15.73 v18.7,15.8 | R18.1 16.38,13.52 v16.2,13.7 | C20.2 C19.2 | C19.2 v25,14 | Y1.P$4 32.4,22.52 C14.1 32.08,21.49 v32.1,21.47 | Y1.P$2 34.33,26.12 C11.2 33.8,27.73 v33.8,28.1 | C17.2 20.52,18.62 20,18.1 20,17.76 v19.84,17.6 | C18.1 23.52,15.29 24.48,15.29 C19.2 | C16.2 33.12,19.12 v33.1,19.1 | D3.2 v27.24,34.1 | C4.2 18.1,33.83 S1.P$2 16.38,33.83 v16.3,33.9 | C15.2 18.24,22 v18.22,22.02 | J103.9 19.72,29 | R9.1 R8.1 R7.1 6.88,29.18 v6.9,29.2
  Top 0.203: U3.7 25.75,21.25 26.4,21.9 | U3.33 30.25,25.25 26.75,21.75 | 25.35,23.25 23.25,25.35 U3.47 23.14,26.61 23.14,26.95 23.02,27.07 C9.2 | 25.35,23.25 26.4,22.2 | U3.54 25.35,23.25 | C12.2 18.8,25.27 C13.2 19.38,24.5 v18.7,24.5 | U3.22 28.25,20.75 v28,20.5 | 12.2,28.8 U2.11 | C7.2 25.96,29 25.16,29.8 24.33,29.8 J103.3
  Top 0.3: X1.GND 6.2,24 v6.5,24.3 | C2.2 6.5,33 U1.2 v8.3,33 | C1.2 11.68,32.2 C3.2 v12.2,32.89 | 26.75,21.75 U3.P$1 26.2,22.3 v26.2,23.5 | 12.2,28.8 U2.15 v11.8,29.3
  Top 0.5: C5.2 C6.2 18.32,29 | C10.2 C8.2 18.32,29 | 19.72,29 18.32,29
  other vias: 16.9,8.6 15.3,10.2 15.3,9.4 16.1,9.4 16.1,10.2 16.1,11 16.9,10.2 16.9,9.4 23.6,11.4 20.9,10.1 20.9,10.9 21.7,8.5 20.9,8.5 21.7,9.3 20.9,9.3 21.7,10.1 21.7,10.9 16.9,11 18,8.9 18,8.1 19.8,8.9 19.8,8.1 29.6,7.9 30.4,7.9 30.4,7.1 29.6,7.1 29.6,8.7 30.4,8.7 30.4,6.3 29.6,6.3 28.9,6.7 28.9,7.5 28.9,8.3 31.1,8.3 31.1,7.5 31.1,6.7 4.3,10.9 5.1,10.9 5.1,10.1 4.3,10.1 4.3,11.7 5.1,11.7 5.1,9.3 4.3,9.3 3.6,9.7 3.6,10.5 3.6,11.3 5.8,11.3 5.8,10.5 5.8,9.7 28,23.5 26,20.5 11.8,28.3 12.8,29.3 12.8,28.3
  pour Bottom (rank 6, no thermals): 36,-1 35.9,-0.9 35.9,14.7 26.9,14.7 25.1,12.9 22.9,12.9 22.9,13.3 25.1,13.3 26.8,15 35.9,15 36,35.5 -1,35.5 -1,-1
  pour Top (rank 3, no thermals): 12.2,11.4 12.2,9.1 10.3,9.1 10.3,8.1 8.6,8.1 8.6,7.2 13.4,7.2 14.3,8.1 17.3,8.1 17.3,11.4
  pour Top (rank 4, no thermals): 20.5,13.4 20.5,5.8 23,5.8 23,9.3 25.2,9.3 25.2,10.4 25.8,11 25.8,13.4
  pour Top (rank 6, no thermals): 35.5,14 26.5,14 26.5,8.5 23.5,5.5 18,5.5 18,-0.5 35.5,-0.5
  pour Top (rank 6, no thermals): -0.5,20 9.3,20 9.3,10.3 7.5,8.5 7.5,7 9,5.5 17,5.5 17,-0.5 -0.5,-0.5
  pour Top (rank 6, no thermals): 17.7,9.5 20.2,9.5 20.2,7.7 17.6,7.7 17.6,9.5
LSSA
  pour Top (rank 4, no thermals): 6.5,10.5 9.4,10.5 10.3,9.6 10.3,9.2 12.1,9.2 12.1,11.4 10.7,11.4 10.3,11.8 6.5,11.8
LSSB
  pour Top (rank 4, no thermals): 28.2,6.2 26,6.2 25.8,6 24,6 24,8 25.8,8 26.3,7.5 28.2,7.5
N$1  (via drill 0.3)
  Top 0.152: R11.2 27,14.36 v26.64,14 | U5.3 0.56,9.88 0.33,10.1 0.33,13.43 0.92,14.02 v1.5,14.02
  Route2 0.152: v26.64,14 25.75,13.11 19.88,13.11 19.76,12.99 17.56,12.99 17.27,12.71 16.51,12.71 16.47,12.74 15.38,12.74 14.69,12.06 14.69,11.88 13.9,11.1 8.07,11.1 4.87,14.3 1.78,14.3 v1.5,14.02
N$2
  Top 0.152: R14.2 30.52,14.26 32.62,14.26 33.89,12.98 33.89,9.59 33.7,9.39 U7.4
N$3  (via drill 0.3)
  Top 0.152: R10.2 v24,14 | v0.61,9.2 1.2,8.61 U5.4
  Route2 0.152: v24,14 23.41,13.41 19.75,13.41 19.63,13.29 17.43,13.29 17.15,13.01 16.63,13.01 16.59,13.05 15.25,13.05 14.39,12.19 14.39,12.01 13.78,11.4 8.2,11.4 5,14.6 1.2,14.6 0.33,13.73 0.33,9.48 v0.61,9.2
N$4  (via drill 0.3)
  Top 0.152: R12.2 28,14.5 v27.5,14 | v1.01,13.29 0.63,12.91 0.63,11.37 0.9,11.1 1.86,11.1 U5.2
  Route2 0.152: v27.5,14 27.09,13.59 27.06,13.59 26.27,12.8 20,12.8 19.88,12.68 17.68,12.68 17.4,12.4 16.38,12.4 16.34,12.44 15.5,12.44 15,11.94 15,11.76 14.03,10.79 7.95,10.79 4.75,13.99 2.29,13.99 1.74,13.44 1.16,13.44 v1.01,13.29
N$5
  Top 0.152: R5.1 26,33.32 27.64,33.32 28.3,33.98 D3.1
N$6  (via drill 0.3)
  Top 0.152: v27,29.9 26.6,30.3 R6.1
  Route2 0.152: v33.8,28.96 34.4,28.36 34.4,27.88 33.82,27.3 29.17,27.3 27,29.47 v27,29.9
  Bottom 0.152: J101.P$16 34.41,7.61 34.5,7.7 34.5,10.2 | 34.5,10.2 34.5,12.7 | 34.5,12.7 34.5,15.2 | 34.5,15.2 34.5,17.7 | 34.5,17.7 34.5,20.3 | 34.5,20.3 34.5,22.8 | 34.5,22.8 34.5,25.3 34.41,25.39 J101.P$9 34.4,26.84 34.4,28.36 v33.8,28.96 | J101.P$10 34.45,22.85 34.5,22.8 | J101.P$11 34.49,20.31 34.5,20.3 | J101.P$12 34.43,17.77 34.5,17.7 | J101.P$13 34.47,15.23 34.5,15.2 | J101.P$14 34.49,12.69 34.5,12.7 | J101.P$15 34.45,10.15 34.5,10.2
N$7
  Top 0.152: R15.2 31.52,15.29 32.45,15.29 34.5,13.24 34.5,7.6 33.76,6.86 U7.2
N$8
  Top 0.152: U7.3 33.83,8.12 34.2,8.49 34.2,13.11 32.53,14.77 R16.2
N$9
  Top 0.152: R4.1 24.8,33.12 D2.1
N$10
  Top 0.152: R2.1 21.3,33.23 D1.1
N$11
  Top 0.152: R9.2 10.08,26.3 10.46,25.92 11.02,25.92 12.2,27.1 13.98,27.1 14.37,27.48 15.16,27.48 U2.2
N$17
  Top 0.152: R19.2 R17.1 30.33,13.73 29.8,14.26 29.52,14.26 R13.2
N$18
  Top 0.152: U2.13 8.72,27.5 R7.2
N$19
  Top 0.152: U2.14 8.57,26.85 8.12,27.3 R8.2
OA1  (via drill 0.3)
  other vias: 9.7,8.6 8.9,8.6 8.9,9.4 9.7,9.4
  pour Route15 (rank 5): 8.5,9.8 8.5,8.4 10.7,6.2 10.7,-0.2 13.8,-0.2 13.8,5.9 9.9,9.8
  pour Top (rank 5, no thermals): 10.1,8.2 10.1,9.6 9.3,10.4 6.5,10.4 6.5,9.3 8.5,9.3 8.5,8.2
OA2  (via drill 0.3)
  other vias: 8.9,12.4 8.1,13.2 7.3,13.2 8.9,13.2
  pour Top (rank 5, no thermals): 6.5,11.9 9.3,11.9 9.3,13.6 6.5,13.6
  pour Route15 (rank 5): 6.9,13.6 6.9,12.7 9.5,10.1 9.9,10.1 14.1,5.9 14.1,-0.2 17.3,-0.2 17.3,6.1 11.9,11.5 11,11.5 9.3,13.2 9.3,13.6
OB1  (via drill 0.3)
  other vias: 25.8,8.5 25,8.8 24.2,8.8 23.4,8.8
  pour Top (rank 5, no thermals): 28.2,7.6 26.4,7.6 25.9,8.1 23,8.1 23,9.3 28.2,9.3
  pour Route15 (rank 5, no thermals): 26.2,9.3 26.2,8.1 24.4,6.3 21.6,6.3 20.6,5.3 20.6,-0.2 17.6,-0.2 17.6,6.1 19.5,8 23,8 23,9.3
OB2  (via drill 0.3)
  other vias: 25.8,5.5 25.8,4.7 26.6,4.7 27.4,4.7
  pour Top (rank 5, no thermals): 28.2,6.1 26.1,6.1 25.9,5.9 25.4,5.9 25.4,4.3 27.8,4.3 27.8,5.1 28.2,5.1
  pour Route15 (rank 5, no thermals): 27.8,6 21.6,6 20.9,5.3 20.9,-0.2 24.2,-0.2 24.2,3.2 25.3,4.3 27.8,4.3
RESET  (via drill 0.3)
  Top 0.152: S1.P$4 18,31.88 C4.1 | C4.1 20,32.88 R1.1 | U3.52 21.87,24.38 21.55,24.38 21.42,24.52 21.42,24.83 21.03,25.22 21.03,26.37 20.89,26.5 17.3,26.5 v17,26.2 | C4.1 19,31.38 19.76,30.62 J103.10
  Route2 0.152: 15.9,26.9 15.9,26.66 16.36,26.2 v17,26.2 | 15.9,26.9 | 15.9,26.9 15.9,30.94 16.24,31.28 17.52,31.28 18.3,30.5 19.7,30.5 J103.10
RTD  (via drill 0.3)
  Top 0.152: R18.2 17.1,12.4 | 17.1,12.4 17.1,11.95 U6.2 | U3.12 28.25,17.12 27.75,16.62 v27.42,16.62 | v16.1,11.86 16.1,12.1 16.4,12.4 17.1,12.4
  Route2 0.152: v27.42,16.62 28.12,15.92 28.12,13.8 27.61,13.28 27.18,13.28 26.4,12.5 21.1,12.5 19.9,11.3 17.6,11.3 17.04,11.86 v16.1,11.86
STOP  (via drill 0.3)
  Top 0.152: U3.44 24.75,27.02 24.52,27.25 24.52,27.57 v24.3,27.8
  Route15 0.152: v23.6,31.6 23.9,31.3 25.14,31.3 25.58,30.87 25.58,28.73 25.14,28.3 24.8,28.3 v24.3,27.8
  Bottom 0.152: v23.6,31.6 23.6,31.96 J3.3
SWDCLK  (via drill 0.3)
  Top 0.152: R3.1 22.26,31.88 J103.4 | v20.73,21.64 21.89,21.64 U3.57
  Route2 0.152: v20.73,21.64 22.74,23.65 24.65,23.65 25.62,24.62 27.38,24.62 28.17,25.4 28.17,27.44 26.01,29.6 25.32,29.6 25.14,29.77 24.36,29.77 J103.4
SWDIO  (via drill 0.3)
  Top 0.152: U3.58 21.94,21.31 21.22,21.31 20.97,21.06 20.36,21.06 v20.23,20.93
  Route2 0.152: v20.23,20.93 20.36,21.06 20.97,21.06 21.31,21.4 21.31,21.79 22.87,23.35 24.78,23.35 25.74,24.31 27.51,24.31 28.47,25.28 28.47,27.57 26.14,29.91 25.5,29.91 J103.2
TERM  (via drill 0.3)
  Top 0.152: U2.5 15.23,29.4 v16.48,29.4 | v25.95,28.07 26.46,28.07 26.63,28.24 27.37,28.24 28.62,26.99 28.62,26.63 U3.36
  Route2 0.152: v16.48,29.4 18.47,27.41 21.65,27.41 22.15,26.91 25.35,26.91 25.95,27.51 v25.95,28.07
USBDM  (via drill 0.3)
  Top 0.152: X1.D- 5.85,25.95 6.2,25.61 17.62,25.61 v17.89,25.88 | v26.72,25.3 26.58,25.3 26.1,25.78 25.62,25.78 25.34,25.5 24.59,25.5 24.25,25.85 U3.45
  Route2 0.152: v26.72,25.3 26.24,25.78 25.62,25.78 25.34,25.5 18.32,25.5 18.23,25.59 18.19,25.59 v17.89,25.88
USBDP  (via drill 0.3)
  Top 0.152: U3.46 23.75,25.75 24.3,25.2 v25.86,25.2 | v17.99,25.01 17.7,25.3 X1.D+
  Route2 0.152: v17.99,25.01 18.18,25.2 v25.86,25.2
VDDCORE
  Top 0.203: 20.56,24.56 21.02,24.1 21.11,24.1 21.46,23.75 U3.53 | 20.56,24.56 C13.1 20.4,24.73 C12.1 | L1.2 19.4,24 19.87,24 20.43,24.56 20.56,24.56
VSENSE  (via drill 0.3)
  Top 0.152: R13.1 v29,16.6 | v27.6,18.6 27.6,18.35 27.25,18 U3.10
  Route2 0.152: v29,16.6 28.7,16.6 27.6,17.7 v27.6,18.6
VSW
  Top 0.203: U3.55 21.05,22.75 L1.1
XIN0
  Top 0.152: U3.31 31.33,25.25 31.7,24.87 33.13,24.87 34,24 Y1.P$1 34,23.07 C14.2
XIN32
  Top 0.152: U3.1 22.35,17.5 Y2.P$1 21.25,16.45 20.8,16.9 20.8,17.48 C17.1
XOUT0
  Top 0.152: U3.32 31.05,25.8 Y1.P$3 33.17,26.57 33.17,26.59 33.27,26.7 C11.1
XOUT32
  Top 0.152: Y2.P$2 21.3,14.12 C18.2 23.25,16.07 U3.2
Y  (via drill 0.3)
  Top 0.152: U2.10 8.45,29.45 8.18,29.18 v8.18,29.16
  Route2 0.152: v8.18,29.16 10.04,29.16 15,24.2 15,16.56 J102.7
Z  (via drill 0.3)
  Top 0.152: U2.12 10.15,28.15 10.65,27.65 10.65,27.23 10.7,27.18 v10.7,26.5
  Route2 0.152: v10.7,26.5 10.7,26 8.5,23.8 8.5,19.5 9.3,18.7 9.3,16.26 J102.8

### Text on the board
bPlace: reset | err | clk | logic pwr | jtag | ucbus | mtm.cba.mit.edu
